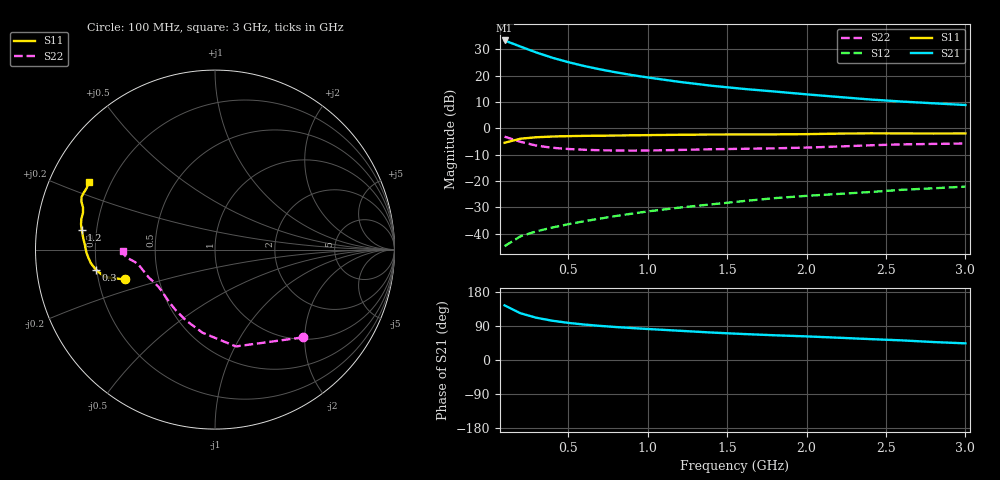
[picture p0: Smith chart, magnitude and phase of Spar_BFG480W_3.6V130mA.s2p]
! Filename: 3_6130BFG480.001
! Title: BFG480W
! Bias: Vce=3.6V; Ic=130mA
! Company: NXP Semiconductors NL
! User: Quality&Reliability T&D
! Measure time: 10 Nov 1999 / 12:01:36
#  MHz  S  MA  R 50
! Freq  S11  S21  S12  S22  :
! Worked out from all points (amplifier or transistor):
!   20 points, 100 MHz to 3 GHz, reference 50 ohm
!   highest |S21| = 33.3 dB at 100 MHz (marker M1)
!   |S21| within 3 dB of that: start of sweep to 230.1 MHz
!   unconditionally stable (mu >= 1): 560.3 MHz to end of sweep
!   at 400 MHz: K = 0.90, MSG = 32.2 dB, |S12| = -37.7 dB
!   at 1.2 GHz: K = 1.10, MAG = 21.9 dB, |S12| = -30.1 dB
!   at 3 GHz: K = 1.06, MAG = 13.9 dB, |S12| = -22.2 dB
!   S11 on the Smith chart (normalised r, x): 100 MHz: 0.31, -0.15; 300 MHz: 0.20, -0.08; 1.2 GHz: 0.14, +0.07; 3 GHz: 0.12, +0.25
100  0.5298 -161.7  46.27 144.2  0.005785 68.4  0.6914 -45.0
200  0.6329 -166.0  35.4 123.3  0.008912 61.2  0.552 -77.8
300  0.6739 -170.5  27.35 111.5  0.01105 61.5  0.4684 -98.5
400  0.6961 -173.8  21.76 103.6  0.01306 63.7  0.4261 -112.5
500  0.7073 -176.4  17.96 98.0  0.01508 66.0  0.4036 -122.3
600  0.7163 -178.6  15.17 93.6  0.01717 68.2  0.3906 -129.5
700  0.7214 179.4  13.12 90.1  0.01929 70.0  0.3823 -135.0
800  0.7267 177.6  11.51 87.0  0.02162 71.5  0.3776 -139.6
900  0.7336 175.8  10.22 84.4  0.02391 73.2  0.3761 -143.5
1000  0.7397 174.3  9.19 81.9  0.02639 74.1  0.3776 -147.0
1200  0.7512 171.4  7.58 77.2  0.03117 75.3  0.3872 -152.6
1400  0.76 169.2  6.411 72.5  0.03591 76.0  0.3992 -156.7
1600  0.764 166.9  5.59 68.6  0.04138 76.6  0.407 -159.9
1800  0.7634 164.4  4.969 65.2  0.04718 76.8  0.416 -163.5
2000  0.7723 162.2  4.396 62.3  0.05209 77.4  0.4292 -167.5
2200  0.7909 160.2  3.921 58.8  0.05665 77.1  0.4497 -171.0
2400  0.7993 158.5  3.512 55.1  0.06159 76.5  0.4744 -173.3
2600  0.7973 156.8  3.207 51.8  0.06784 75.6  0.4941 -174.7
2800  0.7928 154.4  2.971 47.4  0.07259 74.2  0.5043 -176.4
3000  0.7976 151.8  2.759 43.9  0.078 73.3  0.5128 -179.2
